(* Logix 5000 AddOnInstructionDefinition export CM1T_MoveHome; software revision 20.00 *)

TYPE CM1T_DriveStatus :
STRUCT
   StatusValue : SINT;   // Indicates status and error type
   StatusValue1 : SINT;   // Additional status values
   In_Position : BOOL;   // Drive is in position and ready to move
   Moving : BOOL;   // Drive is currently moving
   Disabled : BOOL;   // Drive is disabled
   Error : BOOL;   // Drive is in an error state
   MoveComplete : BOOL;   // Move Complete
   NewStartRequired : BOOL;   // New setpoint required
   HomeAchieved : BOOL;   // Home achieved
END_STRUCT
END_TYPE

TYPE CM1T_Controlword :
STRUCT
   Start : BOOL;   // Start a motion or set a new setpoint
   Halt : BOOL;   // Halt the current motion
   Relative_Move : BOOL;   // Execute the position profile as a relative move
   Speed_Control : BOOL;   // Execute the profile as speed control only
   Disable : BOOL;   // Disable the drive (zero torque)
   Reset_Error : BOOL;   // Reset any existing errors with rising edge
   Set_to_Zero : BOOL;   // Set the current position to 0
   Home : BOOL;   // Execute a home search
END_STRUCT
END_TYPE

TYPE CM1T_Axis :
STRUCT
   Input : SINT[32];   // Data coming from the CM1-T
   Output : SINT[20];   // Data going to the CM1-T
   us50Counter : DINT;   // Controller 50us counter
   ClearCounter : BOOL;
   ModeOfOperation : SINT;   // Type of motion control mode
   ModeOfOperationDisplay : SINT;   // Indicates the active control mode
   Controlword : CM1T_Controlword;   // Controls the drive operation
   DriveStatus : CM1T_DriveStatus;   // Shows status of the drive
   PositionTarget : DINT;   // Final target position for position move
   SpeedTarget : DINT;   // Maximum speed for target move
   TorqueTarget : INT;   // Max torque allowed in 0.1% of peak. Typically 1100
   AccelerationTarget : INT;   // Acceleration for profile move
   DecelerationTarget : INT;   // Deceleration for profile move
   PositionActual : DINT;   // Actual position of the drive
   TargetActual : DINT;   // 1ms position target
   PositionError : DINT;   // Error between the current drive position and the instantaneous target position
   SpeedActual : DINT;   // Actual speed of the drive
   CurrentActual : INT;   // 0.1% of rated current
   OverloadActual : INT;   // 0.1% of overload torque
   DCVoltage : INT;   // DC voltage bus. 0.1V unit
   AnalogIN : INT;   // Value of 10bit analog input
   DigitalIN : SINT;   // Read the digital inputs
   DigitalOUT : SINT;   // Set the digital outputs
   Temperature : SINT;   // Temperature of the drive
   ErrorCode : SINT;   // Indicates error in Ethernet/IP module
END_STRUCT
END_TYPE

ADD_ON_INSTRUCTION CM1T_MoveHome   (* revision 1.0, ExecuteEnableInFalse *)
// Homing Routine
VAR_IN_OUT
   CM1T_Axis : CM1T_Axis; {required}
END_VAR
VAR
   storage_RunHome : BOOL; {access None}
   output_RunHome : BOOL; {access None}
END_VAR

ROUTINE EnableInFalse   (* ladder *)
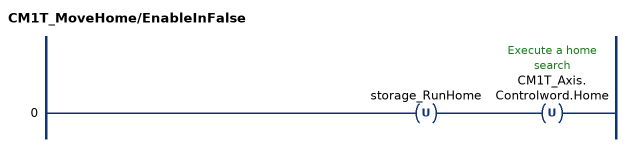
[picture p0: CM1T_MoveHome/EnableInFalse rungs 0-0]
   0: OTU(storage_RunHome)OTU(CM1T_Axis.Controlword.Home);
END_ROUTINE

ROUTINE Logic   (* ladder *)
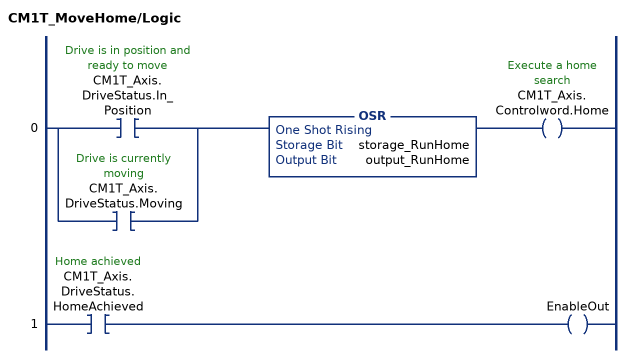
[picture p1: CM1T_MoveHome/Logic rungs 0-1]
   0: [XIC(CM1T_Axis.DriveStatus.In_Position) ,XIC(CM1T_Axis.DriveStatus.Moving) ]OSR(storage_RunHome,output_RunHome)OTE(CM1T_Axis.Controlword.Home);
   1: XIC(CM1T_Axis.DriveStatus.HomeAchieved)OTE(EnableOut);
END_ROUTINE
END_ADD_ON_INSTRUCTION
